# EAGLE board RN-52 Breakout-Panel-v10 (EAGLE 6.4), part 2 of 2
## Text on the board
Bottom: V10 | V10 | V10 | V10 | V10 | V10 | V10 | V10
Dimension: ROUTE OUT | ROUTE OUT | ROUTE OUT | ROUTE OUT | ROUTE OUT | ROUTE OUT | ROUTE OUT | ROUTE OUT | ROUTE OUT | ROUTE OUT | ROUTE OUT
tPlace: SPK_L+ | SPK_L+ | SPK_L+ | SPK_L+ | GPIO3 | GPIO3 | GPIO3 | GPIO3 | SPK_R+ | SPK_R+ | SPK_R+ | SPK_R+ | GPIO2 | GPIO2 | GPIO2 | GPIO2 | SPK_L- | SPK_L- | SPK_L- | SPK_L- | ACI0 | ACI0 | ACI0 | ACI0 | SPK_R- | SPK_R- | SPK_R- | SPK_R- | GPIO4 | GPIO4 | GPIO4 | GPIO4 | GPIO5 | MIC_R- | GPIO5 | MIC_R- | GPIO5 | MIC_R- | GPIO5 | MIC_R- | GPIO12 | MIC_L- | GPIO12 | MIC_L- | GPIO12 | MIC_L- | GPIO12 | MIC_L- | GPIO13 | MIC_R+ | GPIO13 | MIC_R+ | GPIO13 | MIC_R+ | GPIO13 | MIC_R+ | GPIO11 | MIC_L+ | GPIO11 | MIC_L+ | GPIO11 | MIC_L+ | GPIO11 | MIC_L+ | GPIO10 | M_BIAS | GPIO10 | M_BIAS | GPIO10 | M_BIAS | GPIO10 | M_BIAS | GPIO9 | LED0 | LED1 | LED0 | GPIO9 | LED0 | LED1 | LED0 | GPIO9 | LED0 | LED1 | LED0 | GPIO9 | LED0 | LED1 | LED0 | USBD- | LED1 | USBD- | LED1 | USBD- | LED1 | USBD- | LED1 | USBD+ | SPI_MOSI | USBD+ | SPI_MOSI | USBD+ | SPI_MOSI | USBD+ | SPI_MOSI | UART_RTS | SPI_CLK | UART_RTS | SPI_CLK | UART_RTS | SPI_CLK | UART_RTS | SPI_CLK | UART_CTS | SPI_MISO | UART_CTS | SPI_MISO | UART_CTS | SPI_MISO | UART_CTS | SPI_MISO | UART_TX | SPI_SS | UART_TX | SPI_SS | UART_TX | SPI_SS | UART_TX | SPI_SS | UART_RX | PCM_IN | UART_RX | PCM_IN | UART_RX | PCM_IN | UART_RX | PCM_IN | GPIO7 | PCM_OUT | GPIO7 | PCM_OUT | GPIO7 | PCM_OUT | GPIO7 | PCM_OUT | GPIO6 | PCM_SYNC | GPIO6 | PCM_SYNC | GPIO6 | PCM_SYNC | GPIO6 | PCM_SYNC | PWR_EN | PCM_CK | PWR_EN | PCM_CK | PWR_EN | PCM_CK | PWR_EN | PCM_CK | RN-52 Breakout | RN-52 Breakout | RN-52 Breakout | RN-52 Breakout | 3.3V | GND | 3.3V | GND | 3.3V | GND | 3.3V | GND | SPK_L+ | SPK_L+ | SPK_L+ | SPK_L+ | GPIO3 | GPIO3 | GPIO3 | GPIO3 | SPK_R+ | SPK_R+ | SPK_R+ | SPK_R+ | GPIO2 | GPIO2 | GPIO2 | GPIO2 | SPK_L- | SPK_L- | SPK_L- | SPK_L- | ACI0 | ACI0 | ACI0 | ACI0 | SPK_R- | SPK_R- | SPK_R- | SPK_R- | GPIO4 | GPIO4 | GPIO4 | GPIO4 | GPIO5 | MIC_R- | GPIO5 | MIC_R- | GPIO5 | MIC_R- | GPIO5 | MIC_R- | GPIO12 | MIC_L- | GPIO12 | MIC_L- | GPIO12 | MIC_L- | GPIO12 | MIC_L- | GPIO13 | MIC_R+ | GPIO13 | MIC_R+ | GPIO13 | MIC_R+ | GPIO13 | MIC_R+ | GPIO11 | MIC_L+ | GPIO11 | MIC_L+ | GPIO11 | MIC_L+ | GPIO11 | MIC_L+ | GPIO10 | M_BIAS | GPIO10 | M_BIAS | GPIO10 | M_BIAS | GPIO10 | M_BIAS | GPIO9 | LED0 | LED1 | LED0 | GPIO9 | LED0 | LED1 | LED0 | GPIO9 | LED0 | LED1 | LED0 | GPIO9 | LED0 | LED1 | LED0 | USBD- | LED1 | USBD- | LED1 | USBD- | LED1 | USBD- | LED1 | USBD+ | SPI_MOSI | USBD+ | SPI_MOSI | USBD+ | SPI_MOSI | USBD+ | SPI_MOSI | UART_RTS | SPI_CLK | UART_RTS | SPI_CLK | UART_RTS | SPI_CLK | UART_RTS | SPI_CLK | UART_CTS | SPI_MISO | UART_CTS | SPI_MISO | UART_CTS | SPI_MISO | UART_CTS | SPI_MISO | UART_TX | SPI_SS | UART_TX | SPI_SS | UART_TX | SPI_SS | UART_TX | SPI_SS | UART_RX | PCM_IN | UART_RX | PCM_IN | UART_RX | PCM_IN | UART_RX | PCM_IN | GPIO7 | PCM_OUT | GPIO7 | PCM_OUT | GPIO7 | PCM_OUT | GPIO7 | PCM_OUT | GPIO6 | PCM_SYNC | GPIO6 | PCM_SYNC | GPIO6 | PCM_SYNC | GPIO6 | PCM_SYNC | PWR_EN | PCM_CK | PWR_EN | PCM_CK | PWR_EN | PCM_CK | PWR_EN | PCM_CK | RN-52 Breakout | RN-52 Breakout | RN-52 Breakout | RN-52 Breakout | 3.3V | GND | 3.3V | GND | 3.3V | GND | 3.3V | GND
bPlace: SPK_L+ | SPK_L+ | SPK_L+ | SPK_L+ | GPIO3 | GPIO3 | GPIO3 | GPIO3 | SPK_R+ | SPK_R+ | SPK_R+ | SPK_R+ | GPIO2 | GPIO2 | GPIO2 | GPIO2 | SPK_L- | SPK_L- | SPK_L- | SPK_L- | ACI0 | ACI0 | ACI0 | ACI0 | SPK_R- | SPK_R- | SPK_R- | SPK_R- | GPIO4 | GPIO4 | GPIO4 | GPIO4 | GPIO5 | MIC_R- | GPIO5 | MIC_R- | GPIO5 | MIC_R- | GPIO5 | MIC_R- | GPIO12 | MIC_L- | GPIO12 | MIC_L- | GPIO12 | MIC_L- | GPIO12 | MIC_L- | GPIO13 | MIC_R+ | GPIO13 | MIC_R+ | GPIO13 | MIC_R+ | GPIO13 | MIC_R+ | GPIO11 | MIC_L+ | GPIO11 | MIC_L+ | GPIO11 | MIC_L+ | GPIO11 | MIC_L+ | GPIO10 | M_BIAS | GPIO10 | M_BIAS | GPIO10 | M_BIAS | GPIO10 | M_BIAS | GPIO9 | LED0 | GPIO9 | LED0 | GPIO9 | LED0 | GPIO9 | LED0 | USBD- | LED1 | USBD- | LED1 | USBD- | LED1 | USBD- | LED1 | USBD+ | SPI_MOSI | USBD+ | SPI_MOSI | USBD+ | SPI_MOSI | USBD+ | SPI_MOSI | UART_RTS | SPI_CLK | UART_RTS | SPI_CLK | UART_RTS | SPI_CLK | UART_RTS | SPI_CLK | UART_CTS | SPI_MISO | UART_CTS | SPI_MISO | UART_CTS | SPI_MISO | UART_CTS | SPI_MISO | UART_TX | SPI_SS | UART_TX | SPI_SS | UART_TX | SPI_SS | UART_TX | SPI_SS | UART_RX | PCM_IN | UART_RX | PCM_IN | UART_RX | PCM_IN | UART_RX | PCM_IN | GPIO7 | PCM_OUT | GPIO7 | PCM_OUT | GPIO7 | PCM_OUT | GPIO7 | PCM_OUT | GPIO6 | PCM_SYNC | GPIO6 | PCM_SYNC | GPIO6 | PCM_SYNC | GPIO6 | PCM_SYNC | PWR_EN | PCM_CK | PWR_EN | PCM_CK | PWR_EN | PCM_CK | PWR_EN | PCM_CK | 3.3V | GND | 3.3V | GND | 3.3V | GND | 3.3V | GND | SPK_L+ | SPK_L+ | SPK_L+ | SPK_L+ | GPIO3 | GPIO3 | GPIO3 | GPIO3 | SPK_R+ | SPK_R+ | SPK_R+ | SPK_R+ | GPIO2 | GPIO2 | GPIO2 | GPIO2 | SPK_L- | SPK_L- | SPK_L- | SPK_L- | ACI0 | ACI0 | ACI0 | ACI0 | SPK_R- | SPK_R- | SPK_R- | SPK_R- | GPIO4 | GPIO4 | GPIO4 | GPIO4 | GPIO5 | MIC_R- | GPIO5 | MIC_R- | GPIO5 | MIC_R- | GPIO5 | MIC_R- | GPIO12 | MIC_L- | GPIO12 | MIC_L- | GPIO12 | MIC_L- | GPIO12 | MIC_L- | GPIO13 | MIC_R+ | GPIO13 | MIC_R+ | GPIO13 | MIC_R+ | GPIO13 | MIC_R+ | GPIO11 | MIC_L+ | GPIO11 | MIC_L+ | GPIO11 | MIC_L+ | GPIO11 | MIC_L+ | GPIO10 | M_BIAS | GPIO10 | M_BIAS | GPIO10 | M_BIAS | GPIO10 | M_BIAS | GPIO9 | LED0 | GPIO9 | LED0 | GPIO9 | LED0 | GPIO9 | LED0 | USBD- | LED1 | USBD- | LED1 | USBD- | LED1 | USBD- | LED1 | USBD+ | SPI_MOSI | USBD+ | SPI_MOSI | USBD+ | SPI_MOSI | USBD+ | SPI_MOSI | UART_RTS | SPI_CLK | UART_RTS | SPI_CLK | UART_RTS | SPI_CLK | UART_RTS | SPI_CLK | UART_CTS | SPI_MISO | UART_CTS | SPI_MISO | UART_CTS | SPI_MISO | UART_CTS | SPI_MISO | UART_TX | SPI_SS | UART_TX | SPI_SS | UART_TX | SPI_SS | UART_TX | SPI_SS | UART_RX | PCM_IN | UART_RX | PCM_IN | UART_RX | PCM_IN | UART_RX | PCM_IN | GPIO7 | PCM_OUT | GPIO7 | PCM_OUT | GPIO7 | PCM_OUT | GPIO7 | PCM_OUT | GPIO6 | PCM_SYNC | GPIO6 | PCM_SYNC | GPIO6 | PCM_SYNC | GPIO6 | PCM_SYNC | PWR_EN | PCM_CK | PWR_EN | PCM_CK | PWR_EN | PCM_CK | PWR_EN | PCM_CK | 3.3V | GND | 3.3V | GND | 3.3V | GND | 3.3V | GND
